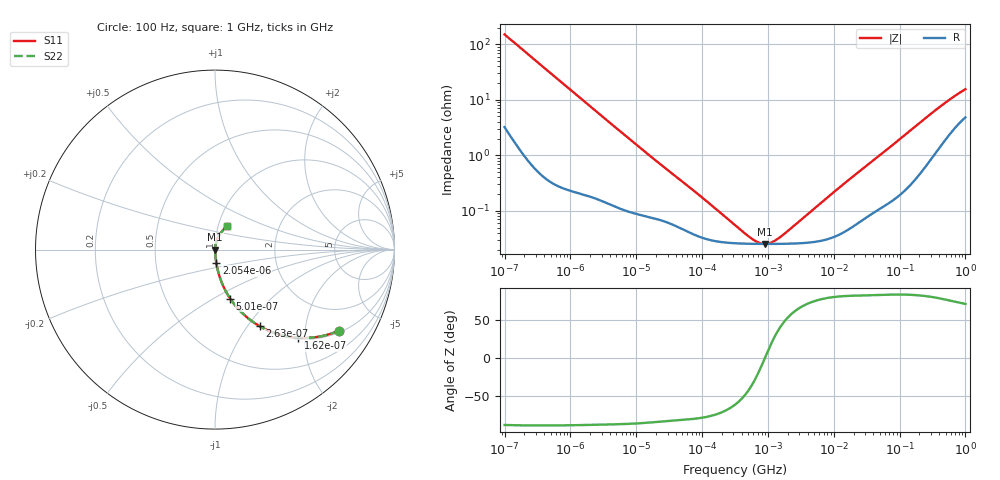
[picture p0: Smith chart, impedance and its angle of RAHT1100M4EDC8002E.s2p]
! RAHT1100M4EDC8002E  S-PARAMETER MODEL  (AEC-Q200 qualified)
! Model Generated by ELNA Corporation (http://www.ty-top.com)
! Version 1.0
! ELNA Control No. 240229
! Copyright (c) 2024 ELNA CO.,LTD. All Rights Reserved.
! Products Name : CONDUCTIVE POLYMER HYBRID ALUMINUM ELECTROLYTIC CAPACITORS
! Characteristics :
!  Capacitance  :  10uF  ,  Rated voltage  :  63V
!  Operating Temp. Range  :  -55 to +105 degC  ,  Endurance  :  10000hr at 105 degC
!  Dimension D  :  6.3mm  ,  Dimension L  :  5.8mm
! Frequency Range : 100Hz - 1GHz
! External Node Assignments :
!  1  o---| |---o  2
# MHz S RI R 50
!Freq[MHz].  S11 Real  S11 Imag  S21 Real  S21 Imag  S12 Real  S12 Imag  S22 Real  S22 Imag
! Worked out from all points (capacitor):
!   401 points, 100 Hz to 1 GHz, reference 50 ohm
!   read as one part in series: C = 10.6 uF near 108 Hz
!   lowest |Z| = 25.3 mohm at 901.6 kHz (marker M1)
!   series resonance near 898.2 kHz, so ESL is about 3 nH
!   S11 on the Smith chart (normalised r, x): 100 Hz: 1.06, -3.00; 162 Hz: 1.03, -1.85; 263 Hz: 1.01, -1.14; 501 Hz: 1.01, -0.60; 2.054 kHz: 1.00, -0.15; 1 GHz: 1.10, +0.29
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0.0001  0.689 -0.4523  0.311 0.4523  0.311 0.4523  0.689 -0.4523
0.000162  0.4621 -0.4913  0.5379 0.4913  0.5379 0.4913  0.4621 -0.4913
0.000263  0.2483 -0.4264  0.7517 0.4264  0.7517 0.4264  0.2483 -0.4264
0.000363  0.1488 -0.3506  0.8512 0.3506  0.8512 0.3506  0.1488 -0.3506
0.000501  0.085 -0.2734  0.915 0.2734  0.915 0.2734  0.085 -0.2734
0.000846  0.0329 -0.1715  0.9671 0.1715  0.9671 0.1715  0.0329 -0.1715
0.001488  0.0121 -0.1  0.9879 0.1  0.9879 0.1  0.0121 -0.1
0.002054  0.00716 -0.0731  0.9928 0.0731  0.9928 0.0731  0.00716 -0.0731
0.005401  0.00192 -0.0284  0.9981 0.0284  0.9981 0.0284  0.00192 -0.0284
0.022131  0.000743 -0.00718  0.9993 0.00718  0.9993 0.00718  0.000743 -0.00718
0.087096  0.000351 -0.00196  0.9996 0.00196  0.9996 0.00196  0.000351 -0.00196
0.316228  0.00026 -0.000486  0.9997 0.000486  0.9997 0.000486  0.00026 -0.000486
0.60256  0.000254 -0.00016  0.9997 0.00016  0.9997 0.00016  0.000254 -0.00016
0.737055  0.000253 -7.79e-05  0.9997 7.79e-05  0.9997 7.79e-05  0.000253 -7.79e-05
0.901571  0.000253 1.48e-06  0.9997 -1.48e-06  0.9997 -1.48e-06  0.000253 1.48e-06
1.148154  0.000253 9.71e-05  0.9997 -9.71e-05  0.9997 -9.71e-05  0.000253 9.71e-05
1.462177  0.000254 0.000198  0.9997 -0.000198  0.9997 -0.000198  0.000254 0.000198
4.704354  0.000272 0.000985  0.9997 -0.000985  0.9997 -0.000985  0.000272 0.000985
69.9842  0.00158 0.0136  0.9984 -0.0136  0.9984 -0.0136  0.00158 0.0136
395.8221  0.0179 0.0691  0.9821 -0.0691  0.9821 -0.0691  0.0179 0.0691
668.3439  0.0396 0.1029  0.9604 -0.1029  0.9604 -0.1029  0.0396 0.1029
1000  0.0645 0.1316  0.9355 -0.1316  0.9355 -0.1316  0.0645 0.1316
